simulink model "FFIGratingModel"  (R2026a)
settings: Solver=ode1  StopTime=T_max  FixedStep=0.00001
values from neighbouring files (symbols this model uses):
  radius = 49    [FFIModelParams_16_02_2021.m]
  t_app = 2    [FFIModelParams_16_02_2021.m]
  t_end = 22    [FFIModelParams_16_02_2021.m]
  t_move = 12    [FFIModelParams_16_02_2021.m]
libraries: LoomingNeuronLibrary x9

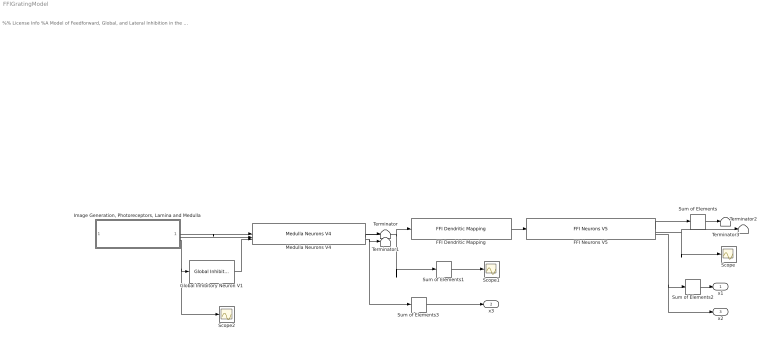
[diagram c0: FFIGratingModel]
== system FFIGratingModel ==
  note: %% License Info %A Model of Feedforward, Global, and Lateral Inhibition in the Locust Visual System. %This model examines the architecture and function of inhibitory mechanisms in the %visual system of locusts, namely those involved in the processing of inputs to a %key looming-sensitive neuron, the lobula giant movement detector (LGMD). %Copyright (c) 2026, Erik Olson, Travis Wiens, and Jack Gray %CITATION: %When using the model code for scientific publications, cite the following work: %Olson EGN, Wiens TK, Gray JR. A model of feedforward, global, and lateral inhibition %in the locust visual system predicts responses to looming stimuli. Biol Cybern. 2021 %Jun;115(3):245-265. doi: 10.1007/s00422-021-00876-8. Epub 2021 May 16. PMID: 33997912. %This program is free software: you can redistribute it and/or modify %it under the terms of the GNU General Public License as published by %the Free Software Foundation, either version 3 of the License, or %(at your option) any later version. %This program is distributed in the hope that it will be useful, %but WITHOUT ANY WARRANTY; without even the implied warranty of %MERCHANTABILITY or FITNESS FOR A PARTICULAR PURPOSE. See the %GNU General Public License for more details. %You should have received a copy of the GNU General Public License %along with this program. If not, see <https://www.gnu.org/licenses/>. %Contact: erik.olson@usask.ca
  FFI Dendritic Mapping : LoomingNeuronLibrary/FFI Dendritic Mapping  r_f=r_field  r_s=r_spacing  pop_FFI=pop_f
  FFI Neurons V5 : LoomingNeuronLibrary/FFI Neurons V5  K_in=K_E_f  g_m=g_L_f  c_m=c  E_rev=E_E  E_rest=E_L  V_t=V_t  Delta_t=Delta_t_f  V_fire=V_fire  tau=tau_alpha_f  g_FFI_adap=Delta_g_A_f  tau_FFI_adap=tau_A_f  E_adap=E_A  g_noise=g_N_f  noise_T=T_noise  pop=pop_f
  Global Inhibitory Neuron V1 : LoomingNeuronLibrary/Global Inhibitory Neuron V1  K_in=K_GI
  "Image Generation, Photoreceptors, Lamina and Medulla" : Subsystem  TreatAsAtomicUnit=on  SystemSampleTime=0.0004
  Medulla Neurons V4 : LoomingNeuronLibrary/Medulla Neurons V4  K_in_ex=K_E_m  K_in_lateral=K_lat_m  K_in_global=K_gl_m  g_m=g_L_m  c_m=c  E_rev_ex=E_E  E_rev_inh=E_I  E_rest=E_L  V_t=V_t  Delta_t=Delta_t_m  V_fire=V_fire  tau=tau_alpha_m  g_med_adap_inc=Delta_g_A_m  tau_med_adap=tau_A_m  E_rev_adap=E_A  g_noise=g_N_m  noise_T=T_noise  radius=radius
  Scope : Scope
  Scope1 : Scope
  Scope2 : Scope
  Sum of Elements{,1..3} (4 alike) : Sum  Inputs=+
  Terminator{,1..3} (4 alike) : Terminator
  x1 : Outport  VectorParamsAs1DForOutWhenUnconnected=off
  x3 : Outport  Port=2  VectorParamsAs1DForOutWhenUnconnected=off
  x2 : Outport  Port=3  VectorParamsAs1DForOutWhenUnconnected=off
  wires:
  "Image Generation, Photoreceptors, Lamina and Medulla"/2(Lateral Inhibition) -> Medulla Neurons V4/2
  Medulla Neurons V4/1 -> Sum of Elements1/1, FFI Dendritic Mapping/1
  Medulla Neurons V4/2 -> Terminator/1
  FFI Dendritic Mapping/1 -> FFI Neurons V5/1
  FFI Neurons V5/2 -> Terminator2/1, Scope/1
  Sum of Elements/1 -> Terminator3/1
  Sum of Elements1/1 -> Scope1/1
  Medulla Neurons V4/3 -> Sum of Elements3/1, Terminator1/1
  FFI Neurons V5/3 -> x2/1, Sum of Elements2/1
  Sum of Elements2/1 -> x1/1
  FFI Neurons V5/1 -> Sum of Elements/1
  Global Inhibitory Neuron V1/1 -> Medulla Neurons V4/3
  "Image Generation, Photoreceptors, Lamina and Medulla"/1(Excitation) -> Medulla Neurons V4/1
  "Image Generation, Photoreceptors, Lamina and Medulla"/3(Global Inhibition) -> Scope2/1, Global Inhibitory Neuron V1/1
  Sum of Elements3/1 -> x3/1

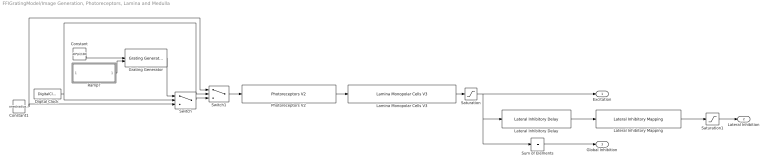
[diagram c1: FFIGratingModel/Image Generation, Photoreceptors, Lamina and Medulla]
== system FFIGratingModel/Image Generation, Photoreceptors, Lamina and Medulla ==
  Constant : Constant  Value=40*pi/180
  Constant1 : Constant  Value=ones(radius*2-1)
  Digital Clock : DigitalClock  SampleTime=-1
  Grating Generator : LoomingNeuronLibrary/Grating Generator  radius=49  theta_max=pi  gratingPeriod=(40*pi/180)/3
  Lamina Monopolar Cells V3 : LoomingNeuronLibrary/Lamina Monopolar Cells V3  K_LMC=K_LMC  gamma_1=b
  Lateral Inhibitory Delay : LoomingNeuronLibrary/Lateral Inhibitory Delay  tau=tau_lat
  Lateral Inhibitory Mapping : LoomingNeuronLibrary/Lateral Inhibitory Mapping  stencil=inhibitory_kernel
  Photoreceptors V2 : LoomingNeuronLibrary/Photoreceptors V2  K_photoD=K_photoD  K_photoP=K_photoP  alpha_1=a_1  alpha_2=a_2
  Ramp? : Subsystem
  Saturation : Saturate  UpperLimit=inf  LowerLimit=0
  Saturation1 : Saturate  UpperLimit=inf  LowerLimit=0
  Sum of Elements : Sum  Inputs=+
  Switch : Switch  Criteria=u2 > Threshold  Threshold=t_app
  Switch1 : Switch  Criteria=u2 > Threshold  Threshold=t_end
  Excitation : Outport  VectorParamsAs1DForOutWhenUnconnected=off
  Lateral Inhibition : Outport  Port=2  VectorParamsAs1DForOutWhenUnconnected=off
  Global Inhibition : Outport  Port=3  VectorParamsAs1DForOutWhenUnconnected=off
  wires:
  Photoreceptors V2/1 -> Lamina Monopolar Cells V3/1
  Lateral Inhibitory Mapping/1 -> Saturation1/1
  Sum of Elements/1 -> Global Inhibition/1
  Digital Clock/1 -> Switch/2, Switch1/2
  Ramp?/1(Out1) -> Grating Generator/2
  Constant/1 -> Grating Generator/1
  Switch1/1 -> Photoreceptors V2/1
  Switch/1 -> Switch1/3
  Constant1/1 -> Switch/3, Switch1/1
  Saturation/1 -> Excitation/1, Lateral Inhibitory Delay/1, Sum of Elements/1
  Grating Generator/1 -> Switch/1
  Lateral Inhibitory Delay/1 -> Lateral Inhibitory Mapping/1
  Lamina Monopolar Cells V3/1 -> Saturation/1
  Saturation1/1 -> Lateral Inhibition/1

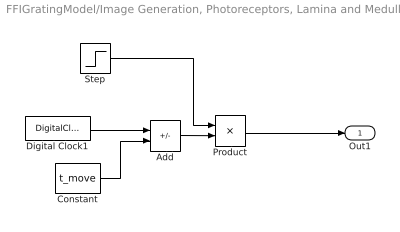
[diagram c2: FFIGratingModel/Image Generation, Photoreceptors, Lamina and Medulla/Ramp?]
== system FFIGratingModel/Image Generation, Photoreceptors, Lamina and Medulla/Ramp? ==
  Add : Sum  Inputs=+-
  Constant : Constant  Value=t_move
  Digital Clock1 : DigitalClock  SampleTime=-1
  Product : Product
  Step : Step  Time=t_move  FinalValue=28.4*pi/180
  Out1 : Outport
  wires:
  Digital Clock1/1 -> Add/1
  Constant/1 -> Add/2
  Add/1 -> Product/2
  Step/1 -> Product/1
  Product/1 -> Out1/1
